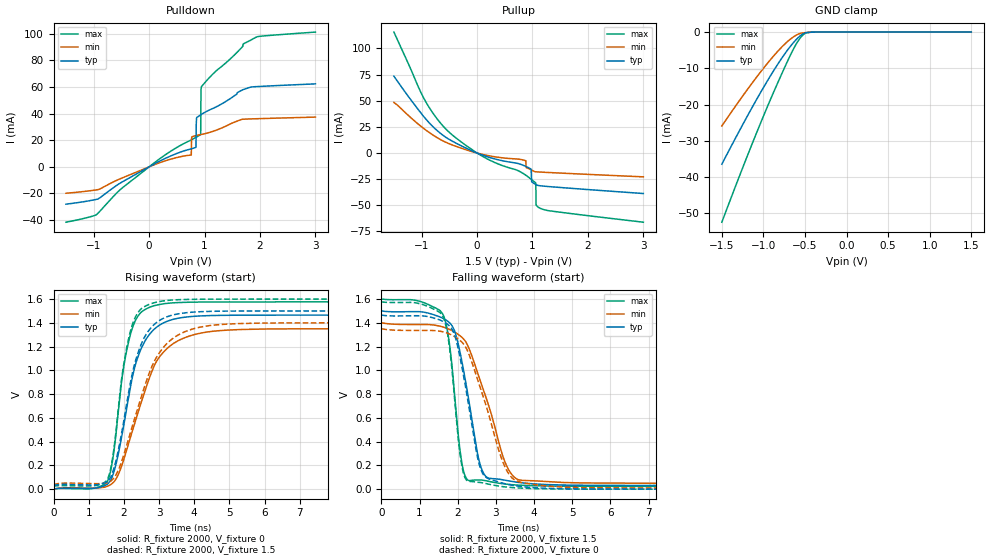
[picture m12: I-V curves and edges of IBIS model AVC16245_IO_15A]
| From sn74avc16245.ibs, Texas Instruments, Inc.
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[Model]   AVC16245_IO_15A
Model_type  I/O
Vinl = 0.49
Vinh = 1.04
Enable   Active-Low
Vref =   0
Rref =   2000
Cref =   30p
Vmeas =   0.75
| variable   typ   min   max
C_comp   6.94pF   6.14pF   7.95pF
| C_pullup   5.32pF   0.74pF   10.43pF
| C_pulldown   8.20pF   1.08pF   26.02pF
| C_tri-state   6.94pF   6.14pF   7.95pF
[Temperature Range]   40   100   -40
| Ambient temperature   25   85   -40
[Voltage range]   1.5   1.4   1.6
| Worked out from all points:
|   slope of the pulldown table from 0 to 0.225 V, typ, clamps not added: 45.2 ohm
|   slope of the pullup table from 0 to 0.225 V, typ, clamps not added: 53.5 ohm
|   GND clamp passes 1 mA (typ) near -0.56 V on its own axis
|   rising waveform, R_fixture 2000, V_fixture 0: 20-80 % time 637ps typ, 920ps min, 437ps max; typ from 0 V to 1.47 V
|   falling waveform, R_fixture 2000, V_fixture 1.5: 20-80 % time 481ps typ, 785ps min, 300ps max; typ from 1.5 V to 0.031 V
|   rising waveform, R_fixture 2000, V_fixture 1.5: 20-80 % time 635ps typ, 945ps min, 433ps max; typ from 0.031 V to 1.5 V
|   falling waveform, R_fixture 2000, V_fixture 0: 20-80 % time 484ps typ, 776ps min, 297ps max; typ from 1.47 V to 0 V
[GND Clamp]
| AVC16245_IO_15A
|   Voltage   I(typ)   I(min)   I(max)
-1.5V     -36.47mA   -25.91mA   -52.48mA
-1.15V    -21.4mA    -14.52mA   -31.68mA
-1V       -15.33mA   -10.01mA   -23.22mA
-865mV    -10.22mA   -6.27mA    -15.95mA
-740mV    -5.914mA   -3.248mA   -9.541mA
-635mV    -2.815mA   -1.258mA   -4.517mA
-570mV    -1.285mA   -459.3uA   -2.031mA
-510mV    -341.5uA   -188.3uA   -518uA
-480mV    -166.9uA   -118.3uA   -185.6uA
-385mV    -13.73uA   -21.91uA   -7.311uA
1.5V      674.1pA    10.89nA    23.96pA
[Pulldown]
| AVC16245_IO_15A
|   Voltage   I(typ)   I(min)   I(max)
-1.5V     -28.04mA   -19.82mA   -41.57mA
-955mV    -24.48mA   -17.33mA   -36.05mA
760mV     13.51mA    8.857mA    20.2mA
770mV     13.63mA    22.38mA    20.42mA
845mV     14.62mA    23.44mA    22.13mA
855mV     36.55mA    23.54mA    22.37mA
925mV     38.88mA    24.16mA    24.13mA
930mV     39.01mA    24.2mA     24.51mA
935mV     39.14mA    24.24mA    57mA
945mV     39.4mA     24.32mA    60.23mA
1.695V    57.93mA    35.74mA    92.16mA
3V        62.27mA    37.32mA    101.2mA
[Pullup]
| AVC16245_IO_15A
|   Voltage   I(typ)   I(min)   I(max)
-1.5V     73.5mA     48.38mA    115.7mA
-980mV    36.08mA    24.24mA    54.47mA
-665mV    19.04mA    13.02mA    28.99mA
15mV      -316.4uA   -207.7uA   -498.7uA
960mV     -14.9mA    -15.65mA   -24.39mA
975mV     -15.34mA   -16.04mA   -25.01mA
985mV     -27.45mA   -16.31mA   -25.43mA
1.055V    -30.1mA    -17.91mA   -28.46mA
1.06V     -30.25mA   -17.93mA   -28.71mA
1.065V    -30.37mA   -17.95mA   -49.69mA
1.1V      -30.94mA   -18.07mA   -51.63mA
3V        -38.73mA   -22.77mA   -66.15mA
[Ramp]
| AVC16245_IO_15A
| variable   typ   min   max
dV/dt_r   0.88/6.40E-10   0.81/9.22E-10   0.95/4.39E-10
dV/dt_f   0.88/4.81E-10   0.82/7.88E-10   0.95/3.10E-10
R_load = 2000
[Rising Waveform]
| AVC16245_IO_15A
R_fixture =   2000
C_fixture =   0
L_fixture =   0
V_fixture =   0
V_fixture_min = 0
V_fixture_max = 0
|   Time   V(typ)   V(min)   V(max)
0s        25.18nV    132.8nV    794.9pV
1.53ns    41.24mV    24.54mV    63.63mV
1.66ns    98.71mV    46.01mV    209.1mV
1.79ns    228mV      93.41mV    504.1mV
1.985ns   518.9mV    238.7mV    1.01V
2.235ns   932.4mV    483.5mV    1.35V
2.625ns   1.259V     849.5mV    1.516V
3.24ns    1.414V     1.187V     1.564V
6.035ns   1.465V     1.348V     1.576V
50ns      1.465V     1.35V      1.576V
[Falling Waveform]
| AVC16245_IO_15A
R_fixture =   2000
C_fixture =   0
L_fixture =   0
V_fixture =   1.5
V_fixture_min = 1.4
V_fixture_max = 1.6
|   Time   V(typ)   V(min)   V(max)
0s        1.5V       1.4V       1.6V
1.625ns   1.436V     1.364V     1.463V
1.795ns   1.397V     1.343V     1.191V
2.095ns   1.096V     1.282V     245.6mV
2.3ns     725.4mV    1.18V      71.84mV
2.535ns   272.8mV    964.1mV    77.74mV
2.7ns     120.7mV    809.3mV    72.94mV
3.27ns    73.54mV    203.7mV    42.34mV
3.715ns   51.89mV    73.44mV    32.08mV
50ns      30.94mV    39.2mV     23.58mV
[Rising Waveform]
| AVC16245_IO_15A
R_fixture =   2000
C_fixture =   0
L_fixture =   0
V_fixture =   1.5
V_fixture_min = 1.4
V_fixture_max = 1.6
|   Time   V(typ)   V(min)   V(max)
0s        30.94mV    39.21mV    23.58mV
1.53ns    63.56mV    54.47mV    79.95mV
1.665ns   129.6mV    77.87mV    237.5mV
1.795ns   264.4mV    131.8mV    542.1mV
1.985ns   554.8mV    277.3mV    1.031V
2.24ns    974.7mV    530mV      1.384V
2.63ns    1.302V     900.8mV    1.543V
3.225ns   1.451V     1.227V     1.588V
5.91ns    1.5V       1.398V     1.6V
50ns      1.5V       1.4V       1.6V
[Falling Waveform]
| AVC16245_IO_15A
R_fixture =   2000
C_fixture =   0
L_fixture =   0
V_fixture =   0
V_fixture_min = 0
V_fixture_max = 0
|   Time   V(typ)   V(min)   V(max)
0s        1.465V     1.35V      1.576V
1.53ns    1.424V     1.329V     1.488V
1.69ns    1.397V     1.317V     1.373V
1.82ns    1.361V     1.301V     1.092V
2.03ns    1.153V     1.259V     371.5mV
2.185ns   895mV      1.207V     99.62mV
2.62ns    153.7mV    824mV      54.63mV
3.3ns     41.23mV    147.2mV    17.06mV
5.455ns   1.275mV    12.01mV    428.8uV
50ns      -3.495uV   -5.676uV   -1.129uV
